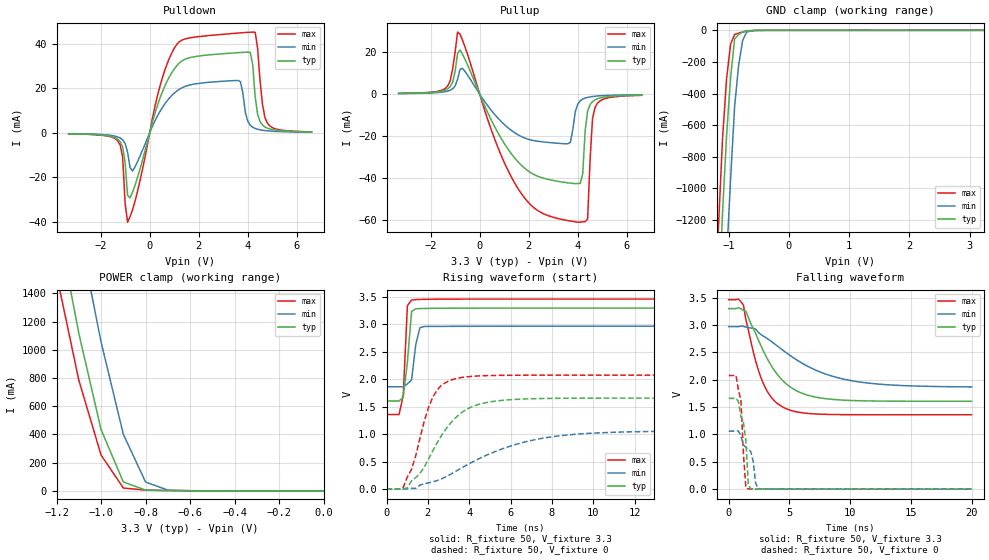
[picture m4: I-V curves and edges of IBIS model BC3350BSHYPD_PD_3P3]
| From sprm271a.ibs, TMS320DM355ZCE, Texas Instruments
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|   GS50 Cell BC3350BSHYPD
|   Model Cell BC3350BSHYPD_PD_3P3
[Model]   BC3350BSHYPD_PD_3P3
Model_type   I/O
Polarity   Non-Inverting
Enable   Active-Low
Vinl =  0.8V
Vinh =  2V
Cref =  15.0000pF
Rref =  100.0000M
Vref =  0V
Vmeas =  1.65
C_comp   0.972592p   0.9599789p   0.9808023p
[Model Spec]
Vinl   0.8V   0.8V   0.8V
Vinh   2V   2V   2V
[Temperature Range]   25   125   -40
[Voltage Range]   3.3   2.97   3.465
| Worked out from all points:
|   slope of the pulldown table from 0 to 0.495 V, typ, clamps not added: 27.8 ohm
|   slope of the pullup table from 0 to 0.495 V, typ, clamps not added: 38.5 ohm
|   GND clamp passes 1 mA (typ) near -0.58 V on its own axis
|   POWER clamp passes 1 mA (typ) near -0.54 V on its own axis
|   rising waveform, R_fixture 50, V_fixture 3.3: 20-80 % time 258ps typ, 248ps min, 156ps max; typ from 1.6 V to 3.3 V
|   rising waveform, R_fixture 50, V_fixture 0: 20-80 % time 1.72ns typ, 3.79ns min, 965ps max; typ from 0 V to 1.66 V
|   falling waveform, R_fixture 50, V_fixture 3.3: 20-80 % time 2.67ns typ, 4.98ns min, 1.72ns max; typ from 3.3 V to 1.6 V
|   falling waveform, R_fixture 50, V_fixture 0: 20-80 % time 548ps typ, 1.01ns min, 327ps max; typ from 1.66 V to 0 V
[POWER_clamp]
|   voltage   I(typ)   I(min)   I(max)
-3.3V     22.25A     22.96A     21.86A
-1.2V     1.942A     2.716A     1.533A
-1.167V   1.667A     2.429A     1.284A
-1.133V   1.392A     2.141A     1.034A
-1.1V     1.117A     1.853A     785.2mA
-1.067V   889.7mA    1.587A     608.1mA
-1.033V   662.1mA    1.321A     431.1mA
-1V       434.5mA    1.055A     254.1mA
-900mV    63.73mA    401.1mA    20.7mA
-800mV    5.777mA    62.83mA    5.256mA
-700mV    2.639mA    5.679mA    3.227mA
-11.55fV  98.21uA    49.4uA     162.3uA
[Pulldown]
|   voltage   I(typ)   I(min)   I(max)
-3.3V     -402.5uA   -328uA     -417.8uA
-1.3V     -2.834mA   -1.803mA   -3.573mA
-1.1V     -6.374mA   -3.139mA   -10.97mA
-900mV    -28.05mA   -8.614mA   -40.19mA
-700mV    -26.75mA   -17.15mA   -34.68mA
400mV     15mA       9.262mA    20.24mA
1.1V      30.16mA    18.8mA     39.75mA
3.7V      36.2mA     23.1mA     45.03mA
4.2V      30.64mA    2.555mA    45.39mA
4.4V      8.36mA     1.642mA    38.05mA
4.8V      2.125mA    940.1uA    4.346mA
6.6V      434.4uA    313.2uA    480.3uA
[Pullup]
|   voltage   I(typ)   I(min)   I(max)
-3.3V     316.4uA    250.6uA    354.6uA
-1.3V     2.461mA    1.426mA    3.872mA
-900mV    19.37mA    6.99mA     29.52mA
-700mV    18.97mA    12.25mA    25.66mA
1.6V      -32.71mA   -19.62mA   -45.68mA
3.6V      -42.27mA   -23.64mA   -60.25mA
4.1V      -42.48mA   -3.206mA   -61.01mA
4.2V      -37.99mA   -2.385mA   -60.84mA
4.4V      -8.156mA   -1.556mA   -59.46mA
4.6V      -3.571mA   -1.147mA   -11.58mA
4.7V      -2.753mA   -1.012mA   -6.453mA
6.6V      -492.8uA   -308.5uA   -611uA
[GND_clamp]
|   voltage   I(typ)   I(min)   I(max)
-3.3V     -22.38A    -23.14A    -21.96A
-1.167V   -1.723A    -2.572A    -1.235A
-1.1V     -1.153A    -1.989A    -682.1mA
-1.033V   -666.4mA   -1.445A    -305.9mA
-966.7mV  -300.1mA   -942.6mA   -87.33mA
-900mV    -54.53mA   -482.6mA   -26.52mA
-833.3mV  -26.34mA   -220.8mA   -17.73mA
-766.7mV  -9.7mA     -63.47mA   -10.39mA
-700mV    -4.621mA   -10.61mA   -4.49mA
-566.7mV  -734.2uA   -1.505mA   -501.8uA
-433.3mV  -74.64uA   -170uA     -70.91uA
3.233V    98.2uA     61.4uA     162.2uA
[Ramp]
| variable   typ   min   max
dV/dt_f   1.026528/2.679218n   0.6686278/5.015857n   1.273867/1.722331n
dV/dt_r   0.995755/1.708729n   0.637017/3.785n   1.246477/0.9557278n
R_load = 50
[Rising Waveform]
R_fixture = 50
V_fixture = 3.3
V_fixture_min = 2.97
V_fixture_max = 3.465
| time   V(typ)   V(min)   V(max)
|   time   V(typ)   V(min)   V(max)
0s        1.605V     1.864V     1.359V
606.1ps   1.605V     1.864V     1.36V
808.1ps   1.672V     1.866V     1.709V
1.01ns    2.316V     1.917V     3.342V
1.212ns   3.235V     1.989V     3.445V
1.414ns   3.286V     2.632V     3.453V
1.616ns   3.289V     2.941V     3.455V
1.818ns   3.291V     2.962V     3.457V
20ns      3.298V     2.969V     3.462V
[Rising Waveform]
R_fixture = 50
V_fixture = 0
V_fixture_min = 0
V_fixture_max = 0
| time   V(typ)   V(min)   V(max)
|   time   V(typ)   V(min)   V(max)
0s        56.69nV    457.1nV    5.317nV
808.1ps   6.317mV    -798.3uV   30.92mV
1.212ns   150.9mV    14.38mV    362.1mV
1.818ns   398mV      95.48mV    1.229V
2.222ns   686.6mV    130.4mV    1.662V
2.626ns   957.6mV    181.2mV    1.881V
3.232ns   1.259V     298.7mV    2.001V
4.848ns   1.578V     619.8mV    2.068V
8.283ns   1.654V     966.9mV    2.076V
20ns      1.658V     1.061V     2.076V
[Falling Waveform]
R_fixture = 50
V_fixture = 3.3
V_fixture_min = 2.97
V_fixture_max = 3.465
| time   V(typ)   V(min)   V(max)
|   time   V(typ)   V(min)   V(max)
0s        3.298V     2.969V     3.462V
808.1ps   3.313V     2.968V     3.472V
1.212ns   3.267V     2.973V     3.362V
2.02ns    2.938V     2.94V      2.512V
2.828ns   2.538V     2.8V       1.943V
3.636ns   2.211V     2.678V     1.643V
4.646ns   1.942V     2.508V     1.478V
6.667ns   1.707V     2.226V     1.381V
9.899ns   1.622V     1.99V      1.361V
20ns      1.605V     1.868V     1.359V
[Falling Waveform]
R_fixture = 50
V_fixture = 0
V_fixture_min = 0
V_fixture_max = 0
| time   V(typ)   V(min)   V(max)
|   time   V(typ)   V(min)   V(max)
0s        1.658V     1.061V     2.076V
606.1ps   1.658V     1.061V     2.076V
1.01ns    1.321V     963.8mV    1.615V
1.212ns   1.22V      809.6mV    655.3mV
1.414ns   889.8mV    763.8mV    25.55mV
1.616ns   85.07mV    725.2mV    4.979mV
1.818ns   9.048mV    691.9mV    2.844mV
2.222ns   2.832mV    109mV      1.372mV
2.626ns   1.652mV    4.176mV    821.6uV
20ns      222.3nV    5.536uV    96.44nV
